(* Logix 5000 AddOnInstructionDefinition export Banner_R95C8UI_Param_v4; software revision 33.00 *)

TYPE Banner_IOL_Port_v4 :   // UDT that has all of the data items necessary to communicate with a specific Port on a IO-Link Master
STRUCT
   Port_Controlled : INT;   // Each bit represents a port on an IO-Link Master. Set to 1 to tell AOI to control that port.
   Port_Activate : INT;   // Each bit represents a port on an IO-Link Master. When ON that port will process any commands in queue.
   Port_Read : INT;   // Each bit represents a port on an IO-Link Master. Used to determine when device AOI has requested a Read command.
   Port_Write : INT;   // Each bit represents a port on an IO-Link Master. Used to determine when device AOI has requested a Write command.
   Port_RW_Complete : INT;   // Each bit represents a port on an IO-Link Master. Tells device AOI that Read or Write request has been completed.
   Port_Device_Read : INT;
   Data_Transfer : SINT[190];   // Array to transfer data from IO-Master to device AOIs.
END_STRUCT
END_TYPE

TYPE Banner_R95C_8UI_MDC_v4 :   // MDC Descriptor parameters for Smart Sensor Profile 2nd edition.
STRUCT
   Lower_Limit : DINT;
   Upper_Limit : DINT;
   Unit : INT;   // 1209 = A, 1240 = V
   Scale : SINT;
END_STRUCT
END_TYPE

TYPE Banner_R95C_8UI_RD_v4 :   // UDT that stores the Read Data for a R95C-8UI-KQ.
STRUCT
   Master_Cycle_Time : INT;
   Min_Cycle_Time : INT;
   M_Sequence_Capability : INT;
   IO_Link_Version_ID : INT;
   Process_Data_Input_Length : INT;
   Process_Data_Output_Length : INT;
   Combined_Vendor_ID : DINT;   // IO-Link Vendor ID
   Vendor_ID1 : INT;
   Vendor_ID2 : INT;
   Combined_Device_ID : DINT;   // IO-Link Device ID
   Device_ID1 : INT;
   Device_ID2 : INT;
   Device_ID3 : INT;
   Serial_Number : STRING;
   All_Time_Run_Time : DINT;
   MDC : Banner_R95C_8UI_MDC_v4[9];
END_STRUCT
END_TYPE

TYPE Banner_R95C_8UI_Setpoints_v4 :   // The Channel setpoints for a R95C-8UI-KQ.
STRUCT
   Voltage_SP1 : DINT;   // Lower limit setpoint.
   Voltage_SP2 : DINT;   // Upper limit setpoint.
   Voltage_Hysteresis : DINT;   // Hysteresis value for the voltage switchpont.
   Current_SP1 : DINT;   // Lower limit setpoint.
   Current_SP2 : DINT;   // Upper limit setpoint.
   Current_Hysteresis : DINT;   // Hysteresis value for the current switchpont.
END_STRUCT
END_TYPE

TYPE Banner_R95C_8UI_v4 :   // All of the parameters for a R95C-8UI-KQ.
STRUCT
   Initial_Global_Read : BOOL;   // Determines if all of the IO-Link data has been read into the PLC yet
   Command : INT;   // Value placed in here will activate a read or write to a specifc IO-Link Index
   Read : Banner_R95C_8UI_RD_v4;   // Read Only Data
   Write : Banner_R95C_8UI_WD_v4;   // Write Data
   Archive : Banner_R95C_8UI_WD_v4;   // Archive of the Write Data
   Reset : BOOL;   // Resets AOI. This will force a complete parameter read of the sensor.
END_STRUCT
END_TYPE

TYPE Banner_R95C_8UI_VSC_v4 :   // Vendor Specific Configuration data elements for a R95C-8UI-KQ.
STRUCT
   PDI_Config : SINT;   // 0 = Analog Value, 1 = Digital Measuring Sensor.
   IOL_Filter_Time : INT;   // Timer to average IOL process data measurement between updates.
   Secondary_Output_Function : SINT;   // 0 = Disabled, 1 = Puse Frequency Modulation.
   PFM_Input_Port : SINT;   // 0 = Analog 1, 1 = Analog 2, 2= Analog 3, 3 = Analog 4, 4 = Analog 5, 5 = Analog 6, 6 = Analog 7, 7 = Analog 8.
   Analog_1_Mode : SINT;   // 0 = Voltage, 1 = Current.
   Analog_2_Mode : SINT;   // 0 = Voltage, 1 = Current.
   Analog_3_Mode : SINT;   // 0 = Voltage, 1 = Current.
   Analog_4_Mode : SINT;   // 0 = Voltage, 1 = Current.
   Analog_5_Mode : SINT;   // 0 = Voltage, 1 = Current.
   Analog_6_Mode : SINT;   // 0 = Voltage, 1 = Current.
   Analog_7_Mode : SINT;   // 0 = Voltage, 1 = Current.
   Analog_8_Mode : SINT;   // 0 = Voltage, 1 = Current.
END_STRUCT
END_TYPE

TYPE Banner_R95C_8UI_WD_v4 :   // UDT that stores the Write Data for a R95C-8UI-KQ.
STRUCT
   System_Command : INT;   // See IODD file for list of commands that can be activated via the System Command interface
   Parameter_Access_Lock : SINT;   // Write access to all parameters is prohibited while value is 1. Only this parameter can be adjusted when value is 1.
   Data_Storage_Lock : SINT;   // Automatic data storage is disabled when this value is equal to 1. Read access is not affected.
   Local_Parameterization_Lock : SINT;   // Parameterization via local control elements on device is disabled.
   Local_User_Interface_Lock : SINT;   // Operation of local user interface is disabled.
   Resettable_Run_Time : DINT;   // Read/Write time counter in hours.
   Near_Freq : DINT;   // 100 to 45000 Hz.
   Far_Freq : DINT;   // 100 to 45000 Hz.
   Pulse_Freq_LOS : DINT;   // 50. Value that the Pulse frequency defaults to when a loss of signal occurs.
   VSC : Banner_R95C_8UI_VSC_v4;
   All_Time_Run_Time_Event_Time : DINT;   // Event indicating the corresponding configured running time has elapsed.
   Resettable_Run_Time_Event_TIme : DINT;   // Running time when an event will be raised indicating that service is required.
   Setpoints : Banner_R95C_8UI_Setpoints_v4[9];
END_STRUCT
END_TYPE

ADD_ON_INSTRUCTION Banner_R95C8UI_Param_v4   (* revision 4.0, vendor Banner Engineering *)
// AOI to read and write parameter data to an IO-Link R95C-8UI-KQ.
VAR_IN_OUT
   R95C : Banner_R95C_8UI_v4; {required}
   Port_Data : Banner_IOL_Port_v4; {required}
END_VAR
VAR_INPUT
   Port : INT; {required}   // Port Number that device is plugged into.
END_VAR
VAR
   Local_Control : DINT; {access None}
   Global_Read_Command_Value : INT; {access None}
   Global_Write_Command_Value : INT; {access None}
   Command_Being_Processed : BOOL; {access None}
   Update_Archive : BOOL; {access None}
   Index_Write_Inprocess : DINT; {access None}
   Index_Write_Control : DINT; {access None}
   Inprocess_Index : DINT; {access None}
   Index1 : DINT; {access None}
   Index2 : DINT; {access None}
   Index3 : DINT; {access None}
   Index_Segment_Read : DINT; {access None}
END_VAR

ROUTINE Logic   (* ladder *)
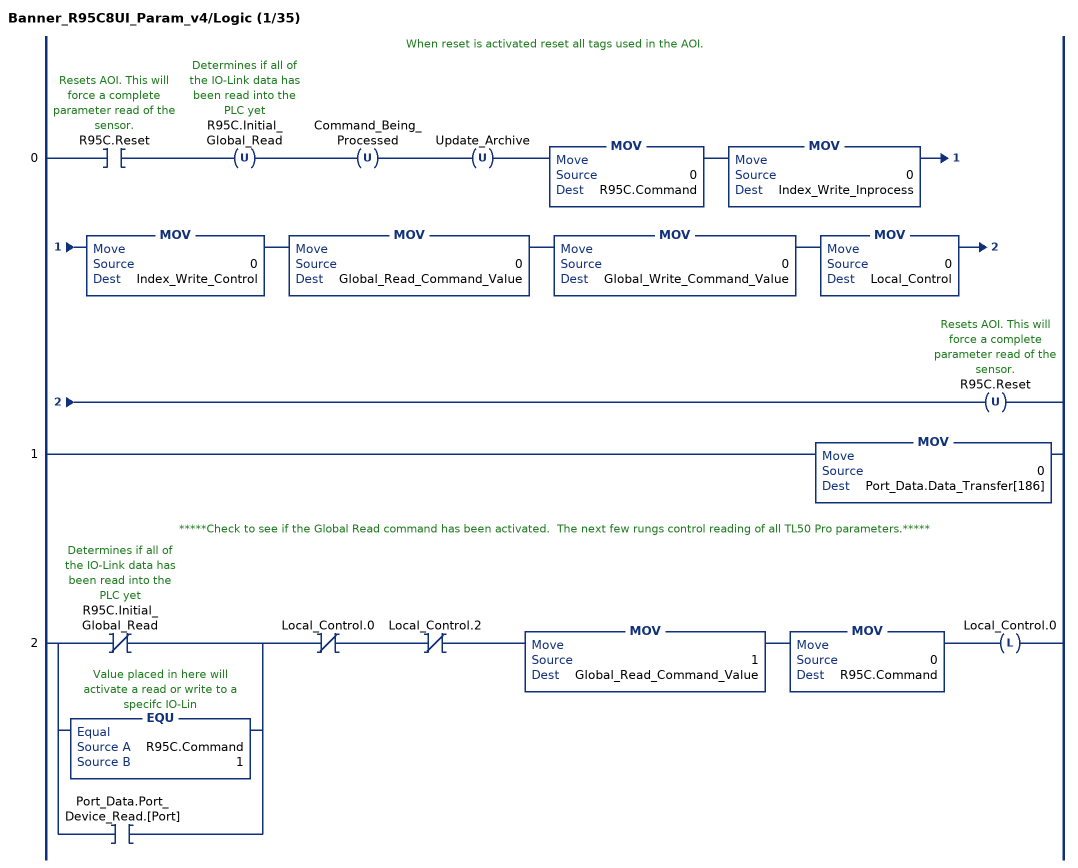
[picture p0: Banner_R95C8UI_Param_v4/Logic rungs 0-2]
   // When reset is activated reset all tags used in the AOI.
   0: XIC(R95C.Reset)OTU(R95C.Initial_Global_Read)OTU(Command_Being_Processed)OTU(Update_Archive)MOV(0,R95C.Command)MOV(0,Index_Write_Inprocess)MOV(0,Index_Write_Control)MOV(0,Global_Read_Command_Value)MOV(0,Global_Write_Command_Value)MOV(0,Local_Control)OTU(R95C.Reset);
   1: MOV(0,Port_Data.Data_Transfer[186]);
   // *****Check to see if the Global Read command has been activated.  The next few rungs control reading of all TL50 Pro parameters.*****
   2: [XIO(R95C.Initial_Global_Read) ,EQU(R95C.Command,1) ,XIC(Port_Data.Port_Device_Read.[Port]) ]XIO(Local_Control.0)XIO(Local_Control.2)MOV(1,Global_Read_Command_Value)MOV(0,R95C.Command)OTL(Local_Control.0);
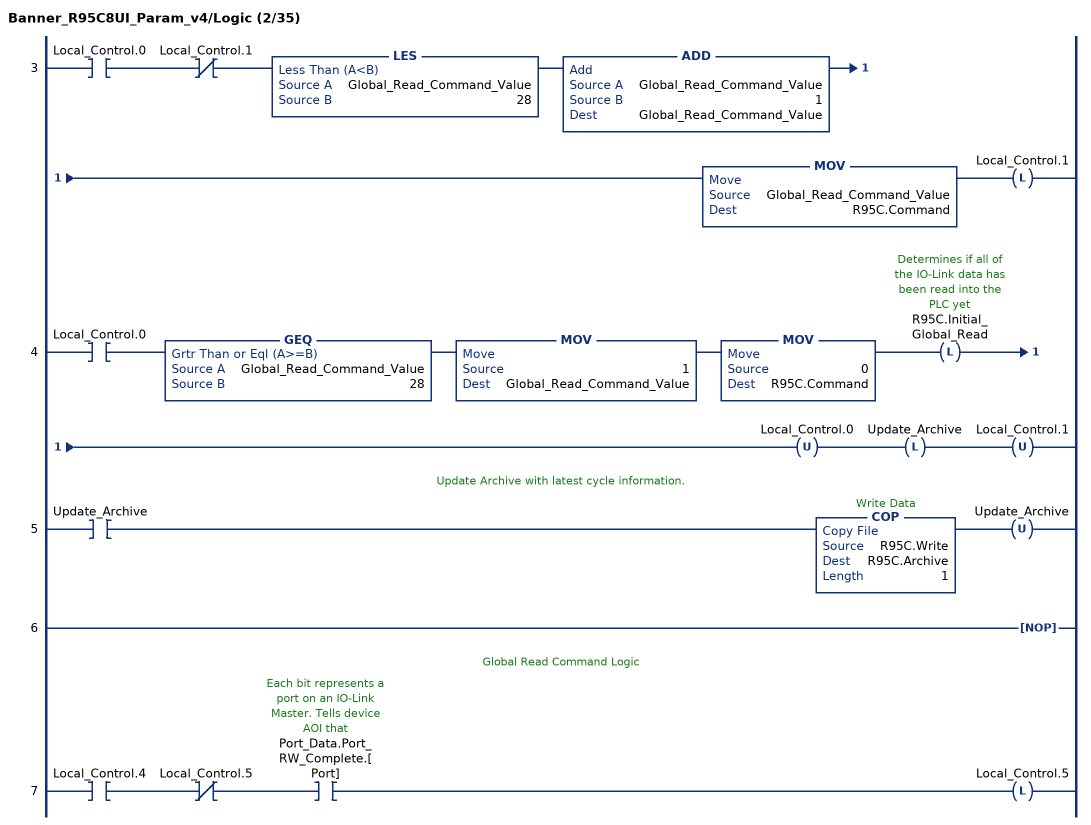
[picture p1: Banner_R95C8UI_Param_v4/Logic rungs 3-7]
   3: XIC(Local_Control.0)XIO(Local_Control.1)LES(Global_Read_Command_Value,28)ADD(Global_Read_Command_Value,1,Global_Read_Command_Value)MOV(Global_Read_Command_Value,R95C.Command)OTL(Local_Control.1);
   4: XIC(Local_Control.0)GEQ(Global_Read_Command_Value,28)MOV(1,Global_Read_Command_Value)MOV(0,R95C.Command)OTL(R95C.Initial_Global_Read)OTU(Local_Control.0)OTL(Update_Archive)OTU(Local_Control.1);
   // Update Archive with latest cycle information.
   5: XIC(Update_Archive)COP(R95C.Write,R95C.Archive,1)OTU(Update_Archive);
   6: NOP();
   // Global Read Command Logic
   7: XIC(Local_Control.4)XIO(Local_Control.5)XIC(Port_Data.Port_RW_Complete.[Port])OTL(Local_Control.5);
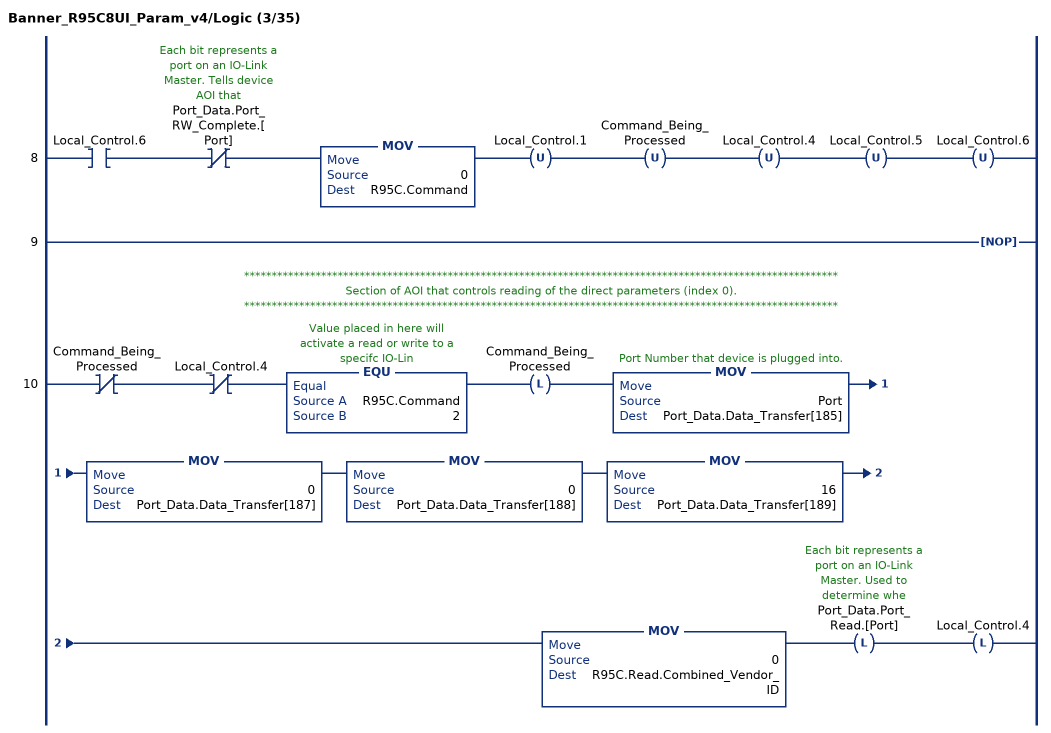
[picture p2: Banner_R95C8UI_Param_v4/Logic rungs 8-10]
   8: XIC(Local_Control.6)XIO(Port_Data.Port_RW_Complete.[Port])MOV(0,R95C.Command)OTU(Local_Control.1)OTU(Command_Being_Processed)OTU(Local_Control.4)OTU(Local_Control.5)OTU(Local_Control.6);
   9: NOP();
   // ************************************************************************************************************
   // Section of AOI that controls reading of the direct parameters (index 0).
   // ************************************************************************************************************
   10: XIO(Command_Being_Processed)XIO(Local_Control.4)EQU(R95C.Command,2)OTL(Command_Being_Processed)MOV(Port,Port_Data.Data_Transfer[185])MOV(0,Port_Data.Data_Transfer[187])MOV(0,Port_Data.Data_Transfer[188])MOV(16,Port_Data.Data_Transfer[189])MOV(0,R95C.Read.Combined_Vendor_ID)OTL(Port_Data.Port_Read.[Port])OTL(Local_Control.4);
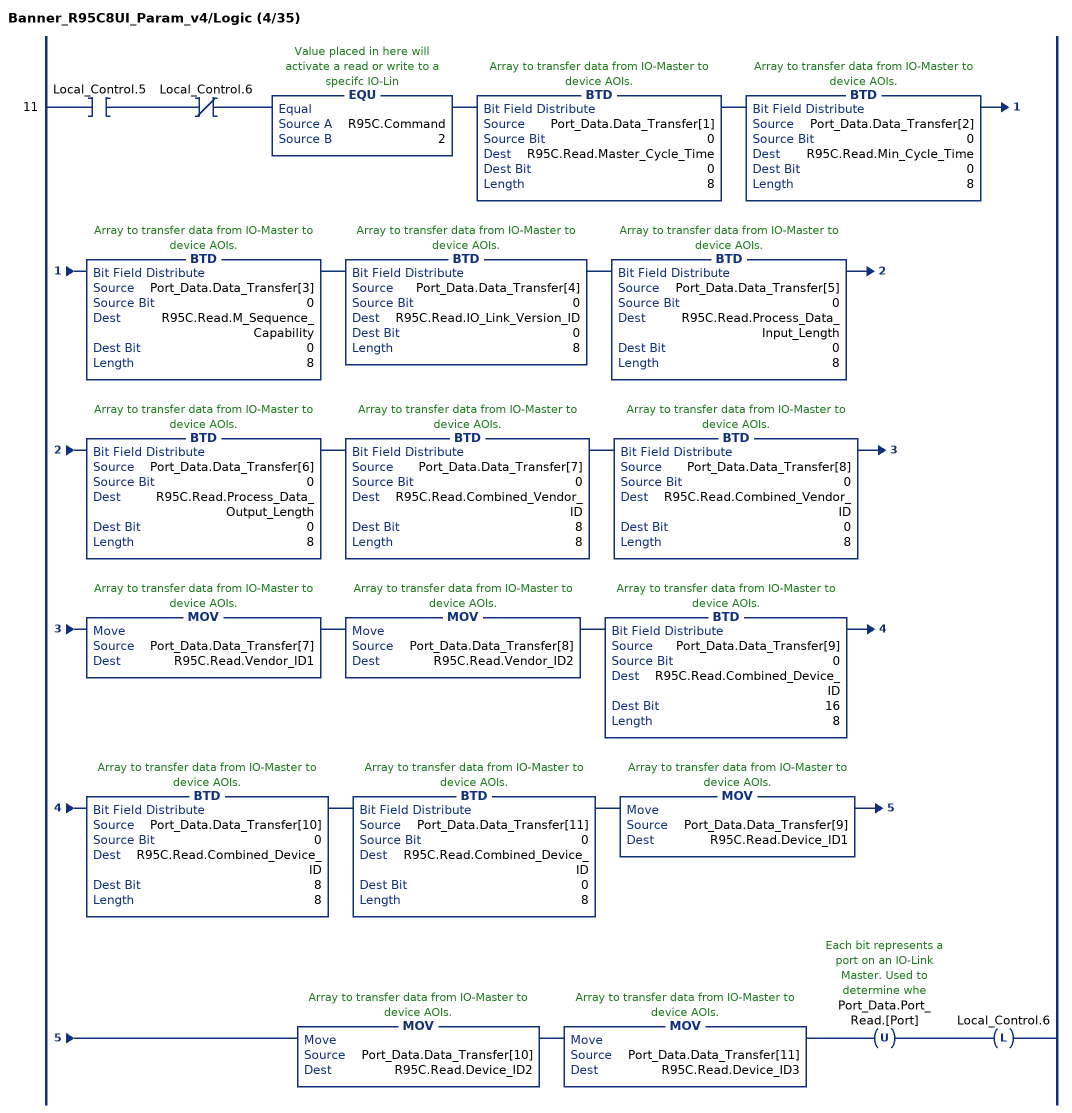
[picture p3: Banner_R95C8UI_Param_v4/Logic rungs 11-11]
   11: XIC(Local_Control.5)XIO(Local_Control.6)EQU(R95C.Command,2)BTD(Port_Data.Data_Transfer[1],0,R95C.Read.Master_Cycle_Time,0,8)BTD(Port_Data.Data_Transfer[2],0,R95C.Read.Min_Cycle_Time,0,8)BTD(Port_Data.Data_Transfer[3],0,R95C.Read.M_Sequence_Capability,0,8)BTD(Port_Data.Data_Transfer[4],0,R95C.Read.IO_Link_Version_ID,0,8)BTD(Port_Data.Data_Transfer[5],0,R95C.Read.Process_Data_Input_Length,0,8)BTD(Port_Data.Data_Transfer[6],0,R95C.Read.Process_Data_Output_Length,0,8)BTD(Port_Data.Data_Transfer[7],0,R95C.Read.Combined_Vendor_ID,8,8)BTD(Port_Data.Data_Transfer[8],0,R95C.Read.Combined_Vendor_ID,0,8)MOV(Port_Data.Data_Transfer[7],R95C.Read.Vendor_ID1)MOV(Port_Data.Data_Transfer[8],R95C.Read.Vendor_ID2)BTD(Port_Data.Data_Transfer[9],0,R95C.Read.Combined_Device_ID,16,8)BTD(Port_Data.Data_Transfer[10],0,R95C.Read.Combined_Device_ID,8,8)BTD(Port_Data.Data_Transfer[11],0,R95C.Read.Combined_Device_ID,0,8)MOV(Port_Data.Data_Transfer[9],R95C.Read.Device_ID1)MOV(Port_Data.Data_Transfer[10],R95C.Read.Device_ID2)MOV(Port_Data.Data_Transfer[11],R95C.Read.Device_ID3)OTU(Port_Data.Port_Read.[Port])OTL(Local_Control.6);
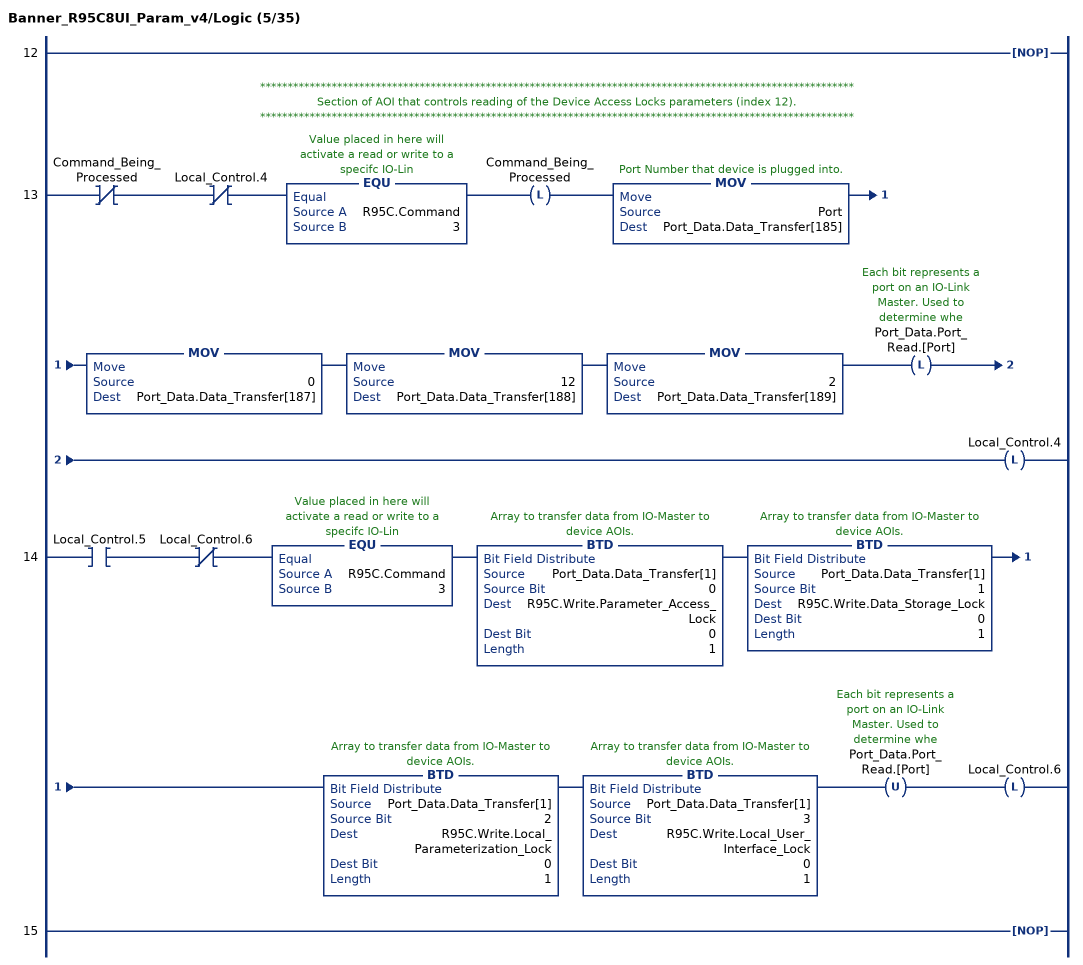
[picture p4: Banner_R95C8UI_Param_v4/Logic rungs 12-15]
   12: NOP();
   // ************************************************************************************************************
   // Section of AOI that controls reading of the Device Access Locks parameters (index 12).
   // ************************************************************************************************************
   13: XIO(Command_Being_Processed)XIO(Local_Control.4)EQU(R95C.Command,3)OTL(Command_Being_Processed)MOV(Port,Port_Data.Data_Transfer[185])MOV(0,Port_Data.Data_Transfer[187])MOV(12,Port_Data.Data_Transfer[188])MOV(2,Port_Data.Data_Transfer[189])OTL(Port_Data.Port_Read.[Port])OTL(Local_Control.4);
   14: XIC(Local_Control.5)XIO(Local_Control.6)EQU(R95C.Command,3)BTD(Port_Data.Data_Transfer[1],0,R95C.Write.Parameter_Access_Lock,0,1)BTD(Port_Data.Data_Transfer[1],1,R95C.Write.Data_Storage_Lock,0,1)BTD(Port_Data.Data_Transfer[1],2,R95C.Write.Local_Parameterization_Lock,0,1)BTD(Port_Data.Data_Transfer[1],3,R95C.Write.Local_User_Interface_Lock,0,1)OTU(Port_Data.Port_Read.[Port])OTL(Local_Control.6);
   15: NOP();
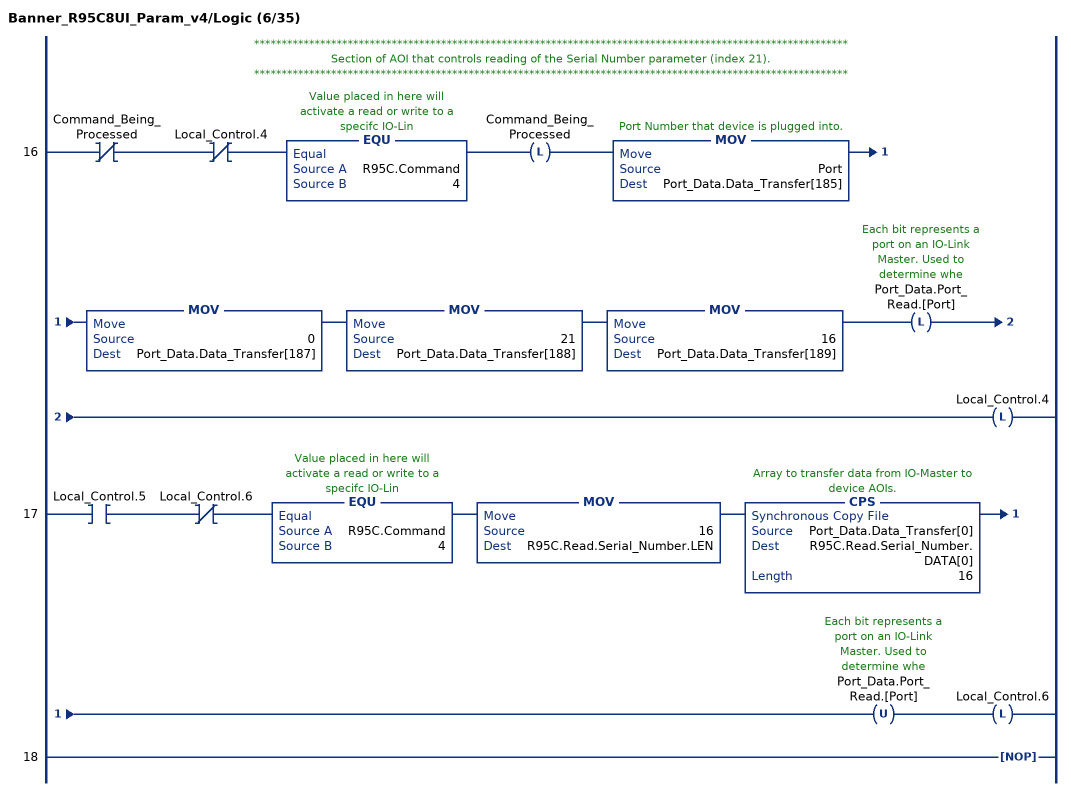
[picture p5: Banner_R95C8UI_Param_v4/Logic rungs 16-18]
   // ************************************************************************************************************
   // Section of AOI that controls reading of the Serial Number parameter (index 21).
   // ************************************************************************************************************
   16: XIO(Command_Being_Processed)XIO(Local_Control.4)EQU(R95C.Command,4)OTL(Command_Being_Processed)MOV(Port,Port_Data.Data_Transfer[185])MOV(0,Port_Data.Data_Transfer[187])MOV(21,Port_Data.Data_Transfer[188])MOV(16,Port_Data.Data_Transfer[189])OTL(Port_Data.Port_Read.[Port])OTL(Local_Control.4);
   17: XIC(Local_Control.5)XIO(Local_Control.6)EQU(R95C.Command,4)MOV(16,R95C.Read.Serial_Number.LEN)CPS(Port_Data.Data_Transfer[0],R95C.Read.Serial_Number.DATA[0],16)OTU(Port_Data.Port_Read.[Port])OTL(Local_Control.6);
   18: NOP();
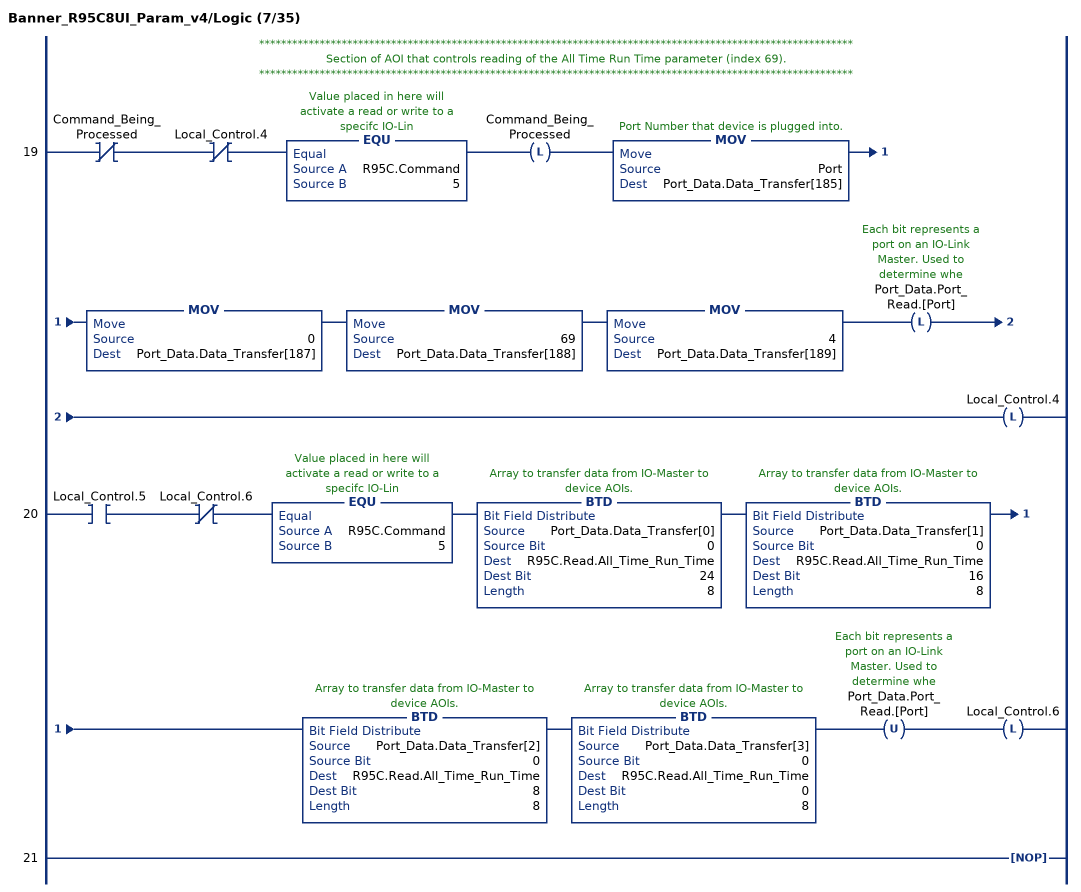
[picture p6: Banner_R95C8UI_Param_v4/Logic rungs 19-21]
   // ************************************************************************************************************
   // Section of AOI that controls reading of the All Time Run Time parameter (index 69).
   // ************************************************************************************************************
   19: XIO(Command_Being_Processed)XIO(Local_Control.4)EQU(R95C.Command,5)OTL(Command_Being_Processed)MOV(Port,Port_Data.Data_Transfer[185])MOV(0,Port_Data.Data_Transfer[187])MOV(69,Port_Data.Data_Transfer[188])MOV(4,Port_Data.Data_Transfer[189])OTL(Port_Data.Port_Read.[Port])OTL(Local_Control.4);
   20: XIC(Local_Control.5)XIO(Local_Control.6)EQU(R95C.Command,5)BTD(Port_Data.Data_Transfer[0],0,R95C.Read.All_Time_Run_Time,24,8)BTD(Port_Data.Data_Transfer[1],0,R95C.Read.All_Time_Run_Time,16,8)BTD(Port_Data.Data_Transfer[2],0,R95C.Read.All_Time_Run_Time,8,8)BTD(Port_Data.Data_Transfer[3],0,R95C.Read.All_Time_Run_Time,0,8)OTU(Port_Data.Port_Read.[Port])OTL(Local_Control.6);
   21: NOP();
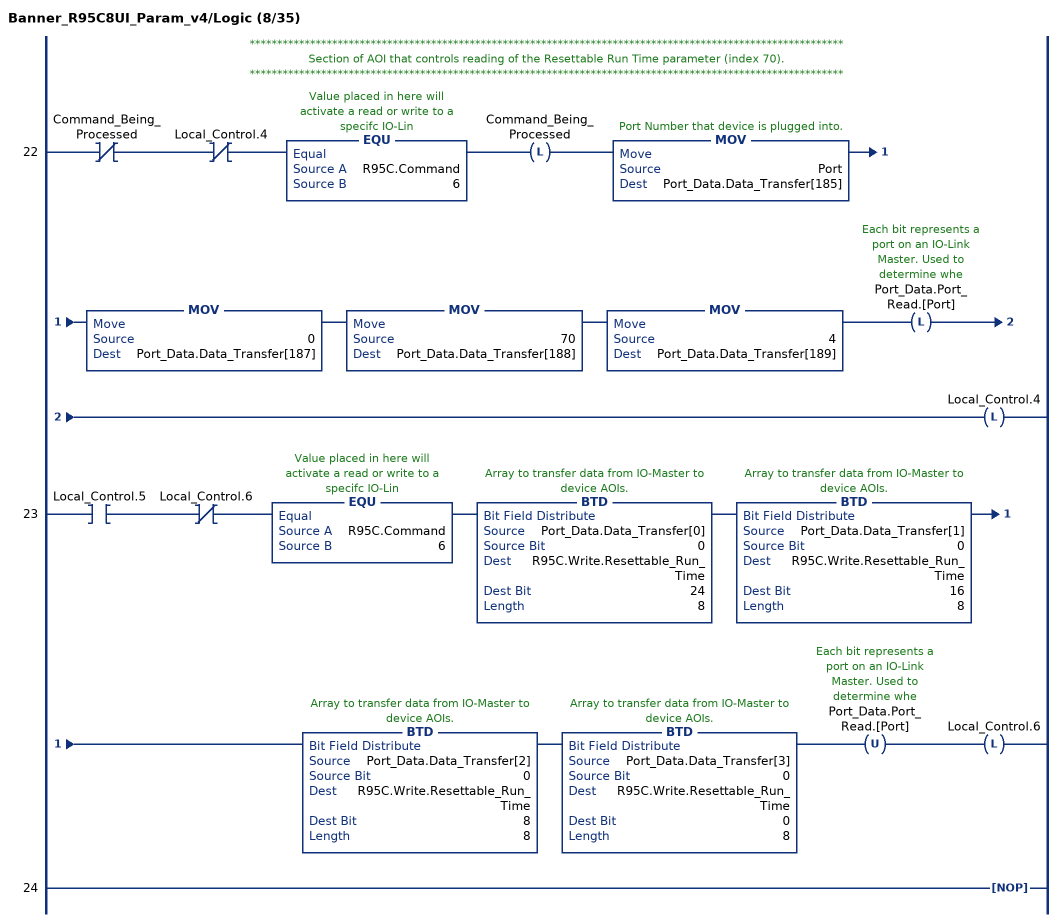
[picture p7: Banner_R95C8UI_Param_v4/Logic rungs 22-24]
   // ************************************************************************************************************
   // Section of AOI that controls reading of the Resettable Run Time parameter (index 70).
   // ************************************************************************************************************
   22: XIO(Command_Being_Processed)XIO(Local_Control.4)EQU(R95C.Command,6)OTL(Command_Being_Processed)MOV(Port,Port_Data.Data_Transfer[185])MOV(0,Port_Data.Data_Transfer[187])MOV(70,Port_Data.Data_Transfer[188])MOV(4,Port_Data.Data_Transfer[189])OTL(Port_Data.Port_Read.[Port])OTL(Local_Control.4);
   23: XIC(Local_Control.5)XIO(Local_Control.6)EQU(R95C.Command,6)BTD(Port_Data.Data_Transfer[0],0,R95C.Write.Resettable_Run_Time,24,8)BTD(Port_Data.Data_Transfer[1],0,R95C.Write.Resettable_Run_Time,16,8)BTD(Port_Data.Data_Transfer[2],0,R95C.Write.Resettable_Run_Time,8,8)BTD(Port_Data.Data_Transfer[3],0,R95C.Write.Resettable_Run_Time,0,8)OTU(Port_Data.Port_Read.[Port])OTL(Local_Control.6);
   24: NOP();
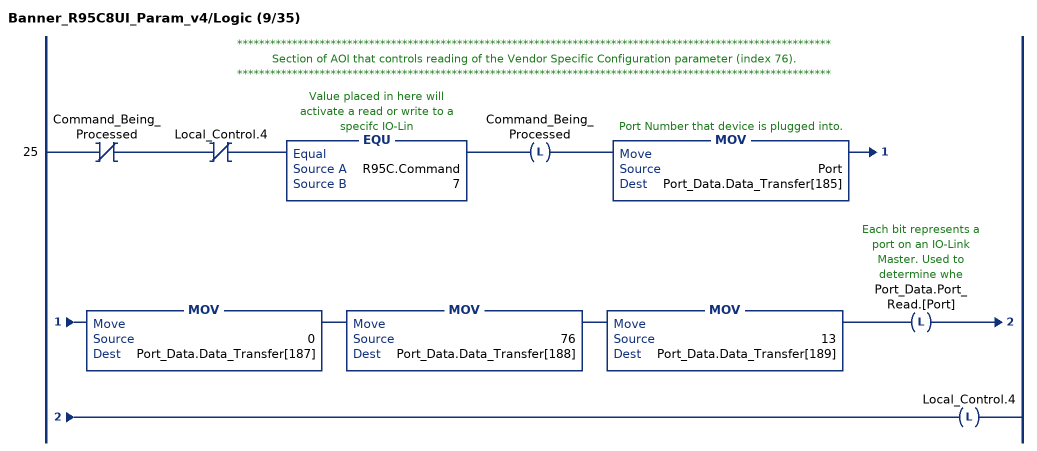
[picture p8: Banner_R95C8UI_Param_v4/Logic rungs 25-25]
   // ************************************************************************************************************
   // Section of AOI that controls reading of the Vendor Specific Configuration parameter (index 76).
   // ************************************************************************************************************
   25: XIO(Command_Being_Processed)XIO(Local_Control.4)EQU(R95C.Command,7)OTL(Command_Being_Processed)MOV(Port,Port_Data.Data_Transfer[185])MOV(0,Port_Data.Data_Transfer[187])MOV(76,Port_Data.Data_Transfer[188])MOV(13,Port_Data.Data_Transfer[189])OTL(Port_Data.Port_Read.[Port])OTL(Local_Control.4);
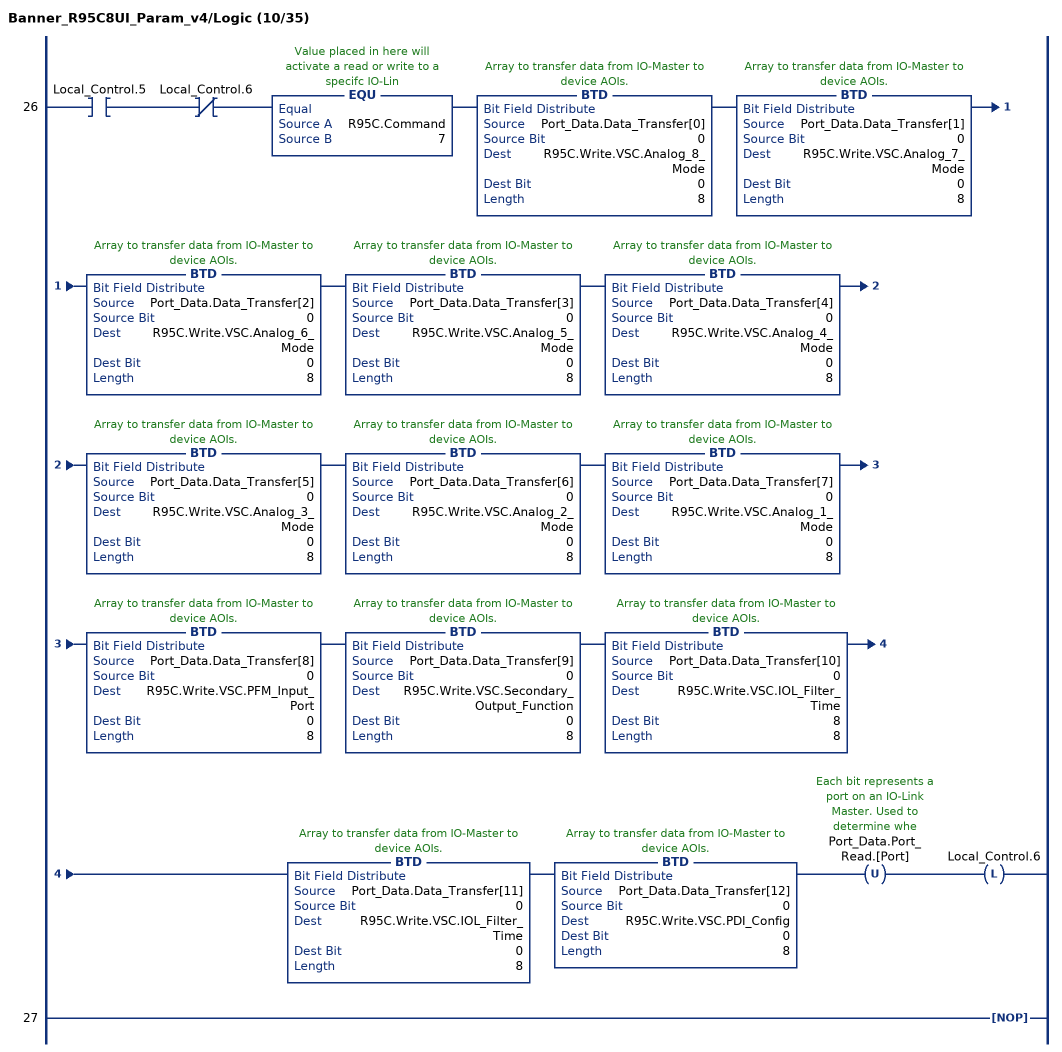
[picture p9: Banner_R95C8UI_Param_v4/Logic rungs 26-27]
   26: XIC(Local_Control.5)XIO(Local_Control.6)EQU(R95C.Command,7)BTD(Port_Data.Data_Transfer[0],0,R95C.Write.VSC.Analog_8_Mode,0,8)BTD(Port_Data.Data_Transfer[1],0,R95C.Write.VSC.Analog_7_Mode,0,8)BTD(Port_Data.Data_Transfer[2],0,R95C.Write.VSC.Analog_6_Mode,0,8)BTD(Port_Data.Data_Transfer[3],0,R95C.Write.VSC.Analog_5_Mode,0,8)BTD(Port_Data.Data_Transfer[4],0,R95C.Write.VSC.Analog_4_Mode,0,8)BTD(Port_Data.Data_Transfer[5],0,R95C.Write.VSC.Analog_3_Mode,0,8)BTD(Port_Data.Data_Transfer[6],0,R95C.Write.VSC.Analog_2_Mode,0,8)BTD(Port_Data.Data_Transfer[7],0,R95C.Write.VSC.Analog_1_Mode,0,8)BTD(Port_Data.Data_Transfer[8],0,R95C.Write.VSC.PFM_Input_Port,0,8)BTD(Port_Data.Data_Transfer[9],0,R95C.Write.VSC.Secondary_Output_Function,0,8)BTD(Port_Data.Data_Transfer[10],0,R95C.Write.VSC.IOL_Filter_Time,8,8)BTD(Port_Data.Data_Transfer[11],0,R95C.Write.VSC.IOL_Filter_Time,0,8)BTD(Port_Data.Data_Transfer[12],0,R95C.Write.VSC.PDI_Config,0,8)OTU(Port_Data.Port_Read.[Port])OTL(Local_Control.6);
   27: NOP();
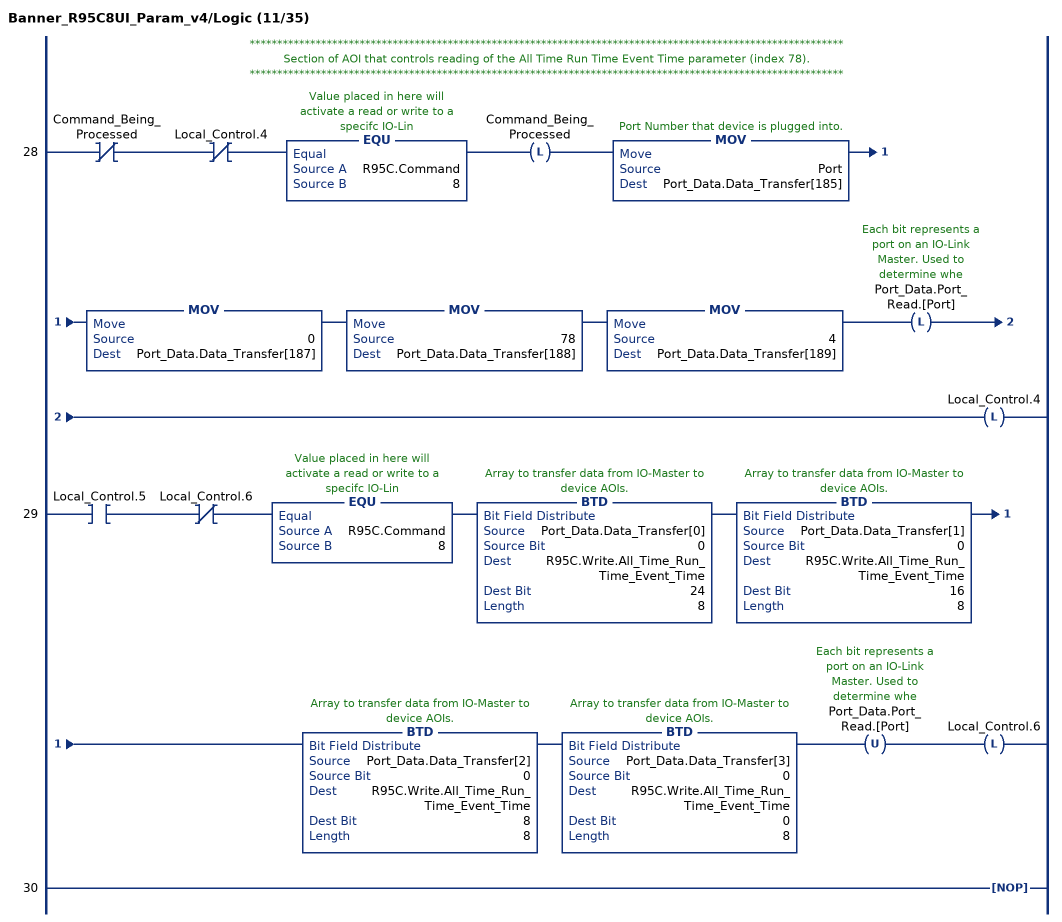
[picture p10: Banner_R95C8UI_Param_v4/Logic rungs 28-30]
   // ************************************************************************************************************
   // Section of AOI that controls reading of the All Time Run Time Event Time parameter (index 78).
   // ************************************************************************************************************
   28: XIO(Command_Being_Processed)XIO(Local_Control.4)EQU(R95C.Command,8)OTL(Command_Being_Processed)MOV(Port,Port_Data.Data_Transfer[185])MOV(0,Port_Data.Data_Transfer[187])MOV(78,Port_Data.Data_Transfer[188])MOV(4,Port_Data.Data_Transfer[189])OTL(Port_Data.Port_Read.[Port])OTL(Local_Control.4);
   29: XIC(Local_Control.5)XIO(Local_Control.6)EQU(R95C.Command,8)BTD(Port_Data.Data_Transfer[0],0,R95C.Write.All_Time_Run_Time_Event_Time,24,8)BTD(Port_Data.Data_Transfer[1],0,R95C.Write.All_Time_Run_Time_Event_Time,16,8)BTD(Port_Data.Data_Transfer[2],0,R95C.Write.All_Time_Run_Time_Event_Time,8,8)BTD(Port_Data.Data_Transfer[3],0,R95C.Write.All_Time_Run_Time_Event_Time,0,8)OTU(Port_Data.Port_Read.[Port])OTL(Local_Control.6);
   30: NOP();
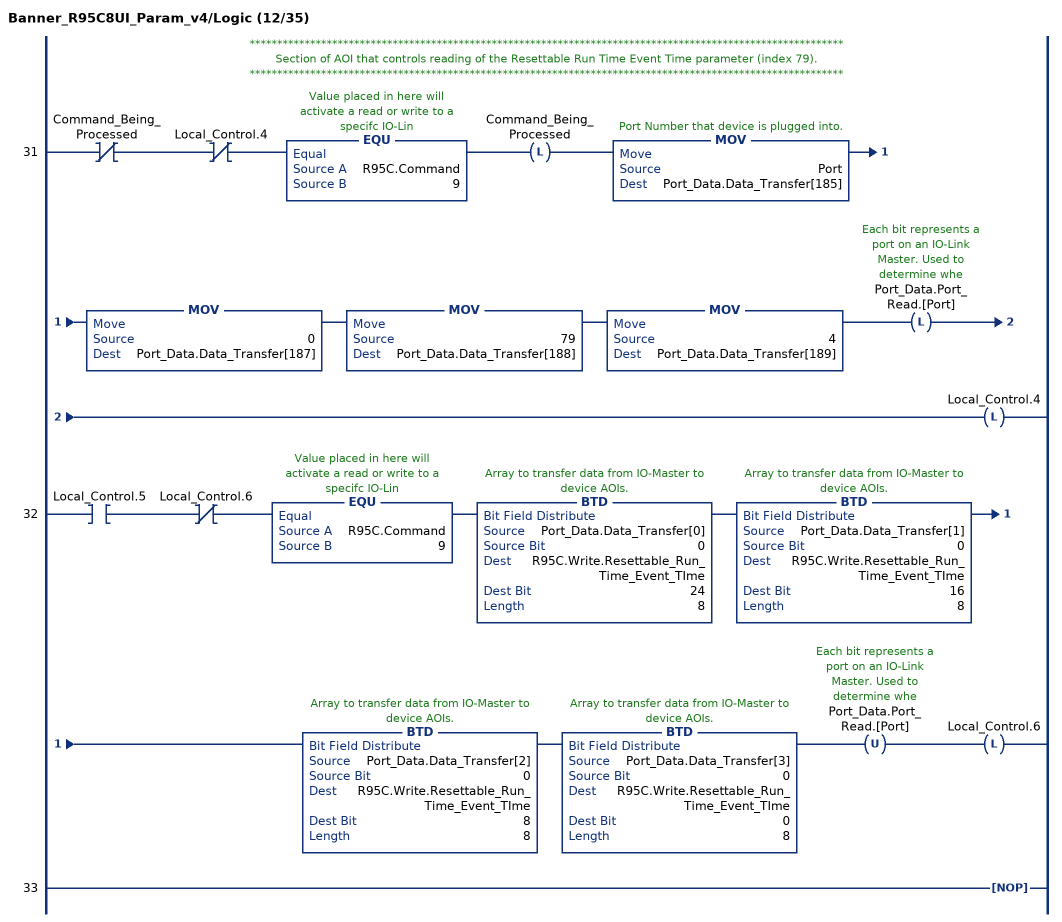
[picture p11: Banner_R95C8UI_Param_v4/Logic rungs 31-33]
   // ************************************************************************************************************
   // Section of AOI that controls reading of the Resettable Run Time Event Time parameter (index 79).
   // ************************************************************************************************************
   31: XIO(Command_Being_Processed)XIO(Local_Control.4)EQU(R95C.Command,9)OTL(Command_Being_Processed)MOV(Port,Port_Data.Data_Transfer[185])MOV(0,Port_Data.Data_Transfer[187])MOV(79,Port_Data.Data_Transfer[188])MOV(4,Port_Data.Data_Transfer[189])OTL(Port_Data.Port_Read.[Port])OTL(Local_Control.4);
   32: XIC(Local_Control.5)XIO(Local_Control.6)EQU(R95C.Command,9)BTD(Port_Data.Data_Transfer[0],0,R95C.Write.Resettable_Run_Time_Event_TIme,24,8)BTD(Port_Data.Data_Transfer[1],0,R95C.Write.Resettable_Run_Time_Event_TIme,16,8)BTD(Port_Data.Data_Transfer[2],0,R95C.Write.Resettable_Run_Time_Event_TIme,8,8)BTD(Port_Data.Data_Transfer[3],0,R95C.Write.Resettable_Run_Time_Event_TIme,0,8)OTU(Port_Data.Port_Read.[Port])OTL(Local_Control.6);
   33: NOP();
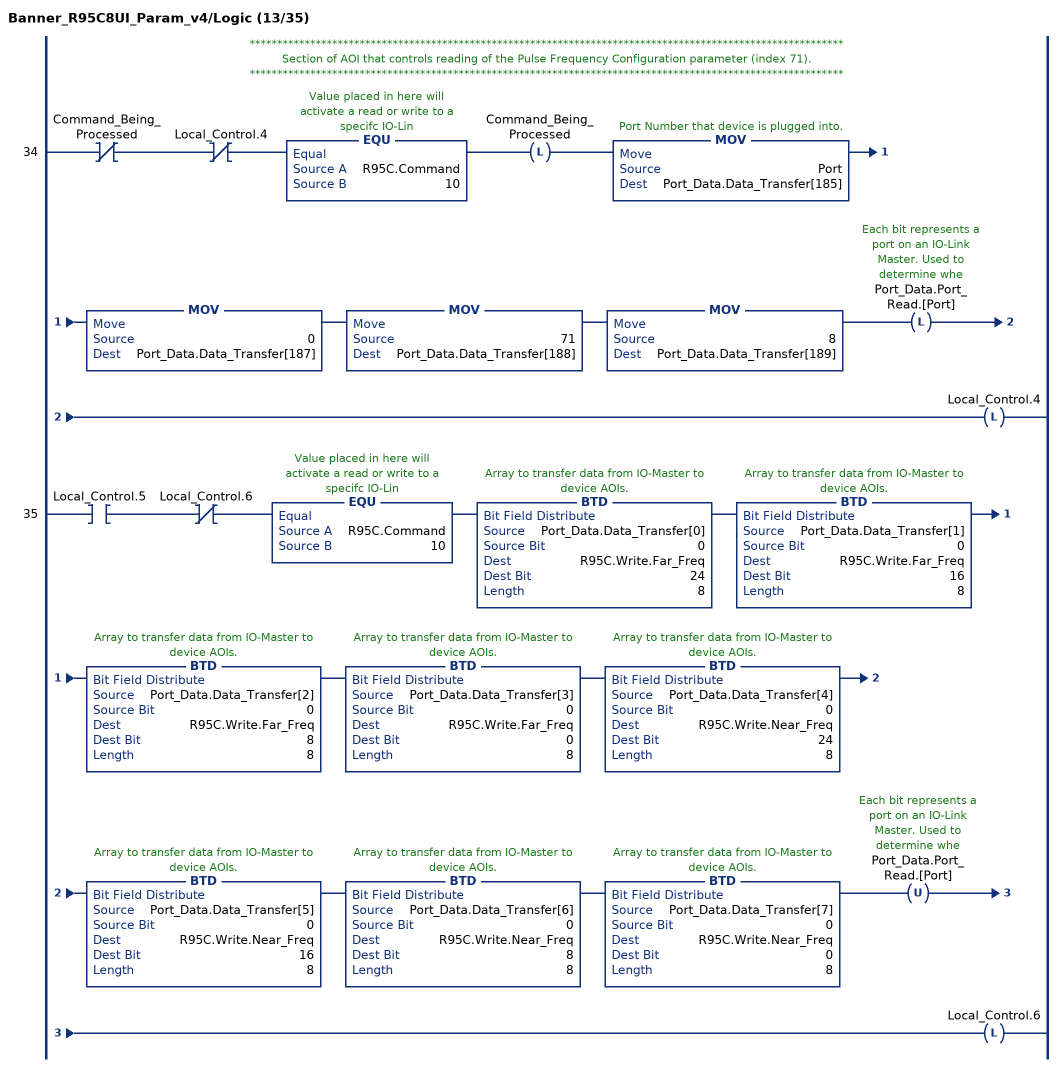
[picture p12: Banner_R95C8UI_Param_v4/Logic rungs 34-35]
   // ************************************************************************************************************
   // Section of AOI that controls reading of the Pulse Frequency Configuration parameter (index 71).
   // ************************************************************************************************************
   34: XIO(Command_Being_Processed)XIO(Local_Control.4)EQU(R95C.Command,10)OTL(Command_Being_Processed)MOV(Port,Port_Data.Data_Transfer[185])MOV(0,Port_Data.Data_Transfer[187])MOV(71,Port_Data.Data_Transfer[188])MOV(8,Port_Data.Data_Transfer[189])OTL(Port_Data.Port_Read.[Port])OTL(Local_Control.4);
   35: XIC(Local_Control.5)XIO(Local_Control.6)EQU(R95C.Command,10)BTD(Port_Data.Data_Transfer[0],0,R95C.Write.Far_Freq,24,8)BTD(Port_Data.Data_Transfer[1],0,R95C.Write.Far_Freq,16,8)BTD(Port_Data.Data_Transfer[2],0,R95C.Write.Far_Freq,8,8)BTD(Port_Data.Data_Transfer[3],0,R95C.Write.Far_Freq,0,8)BTD(Port_Data.Data_Transfer[4],0,R95C.Write.Near_Freq,24,8)BTD(Port_Data.Data_Transfer[5],0,R95C.Write.Near_Freq,16,8)BTD(Port_Data.Data_Transfer[6],0,R95C.Write.Near_Freq,8,8)BTD(Port_Data.Data_Transfer[7],0,R95C.Write.Near_Freq,0,8)OTU(Port_Data.Port_Read.[Port])OTL(Local_Control.6);
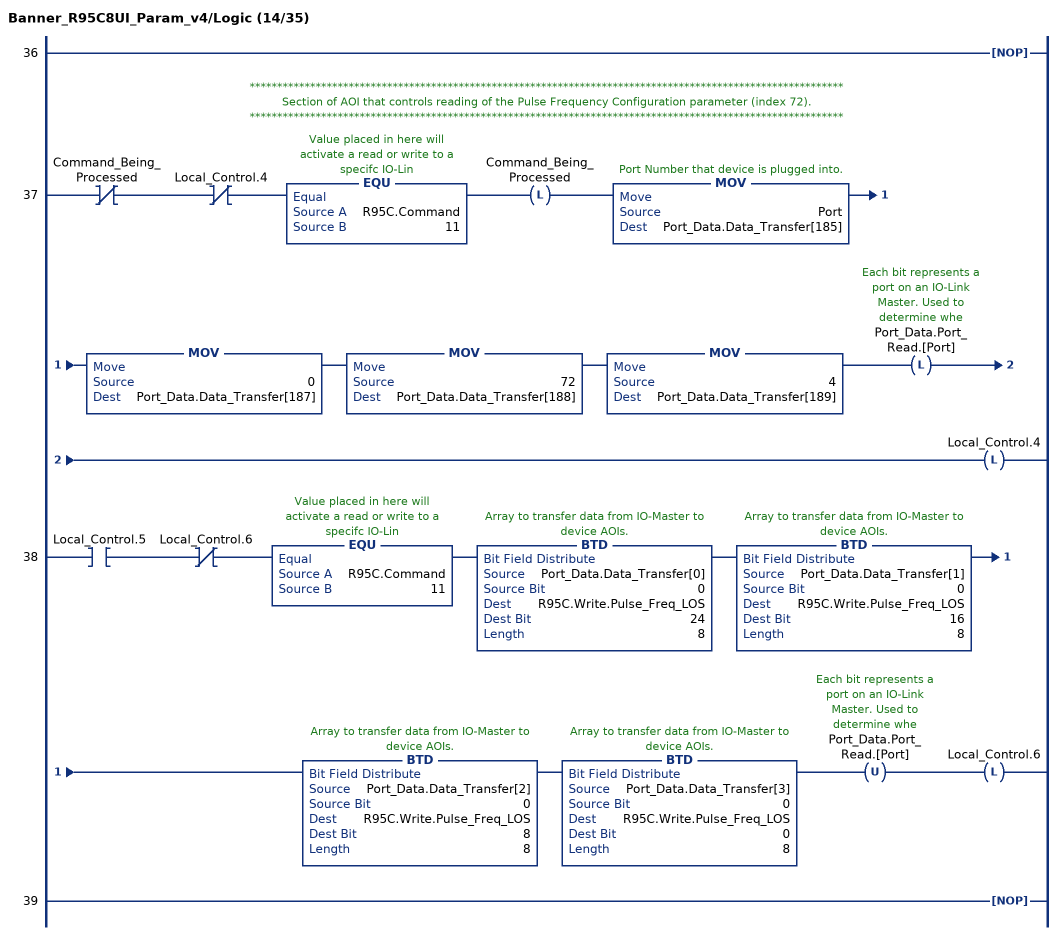
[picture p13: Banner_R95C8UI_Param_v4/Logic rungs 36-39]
   36: NOP();
   // ************************************************************************************************************
   // Section of AOI that controls reading of the Pulse Frequency Configuration parameter (index 72).
   // ************************************************************************************************************
   37: XIO(Command_Being_Processed)XIO(Local_Control.4)EQU(R95C.Command,11)OTL(Command_Being_Processed)MOV(Port,Port_Data.Data_Transfer[185])MOV(0,Port_Data.Data_Transfer[187])MOV(72,Port_Data.Data_Transfer[188])MOV(4,Port_Data.Data_Transfer[189])OTL(Port_Data.Port_Read.[Port])OTL(Local_Control.4);
   38: XIC(Local_Control.5)XIO(Local_Control.6)EQU(R95C.Command,11)BTD(Port_Data.Data_Transfer[0],0,R95C.Write.Pulse_Freq_LOS,24,8)BTD(Port_Data.Data_Transfer[1],0,R95C.Write.Pulse_Freq_LOS,16,8)BTD(Port_Data.Data_Transfer[2],0,R95C.Write.Pulse_Freq_LOS,8,8)BTD(Port_Data.Data_Transfer[3],0,R95C.Write.Pulse_Freq_LOS,0,8)OTU(Port_Data.Port_Read.[Port])OTL(Local_Control.6);
   39: NOP();
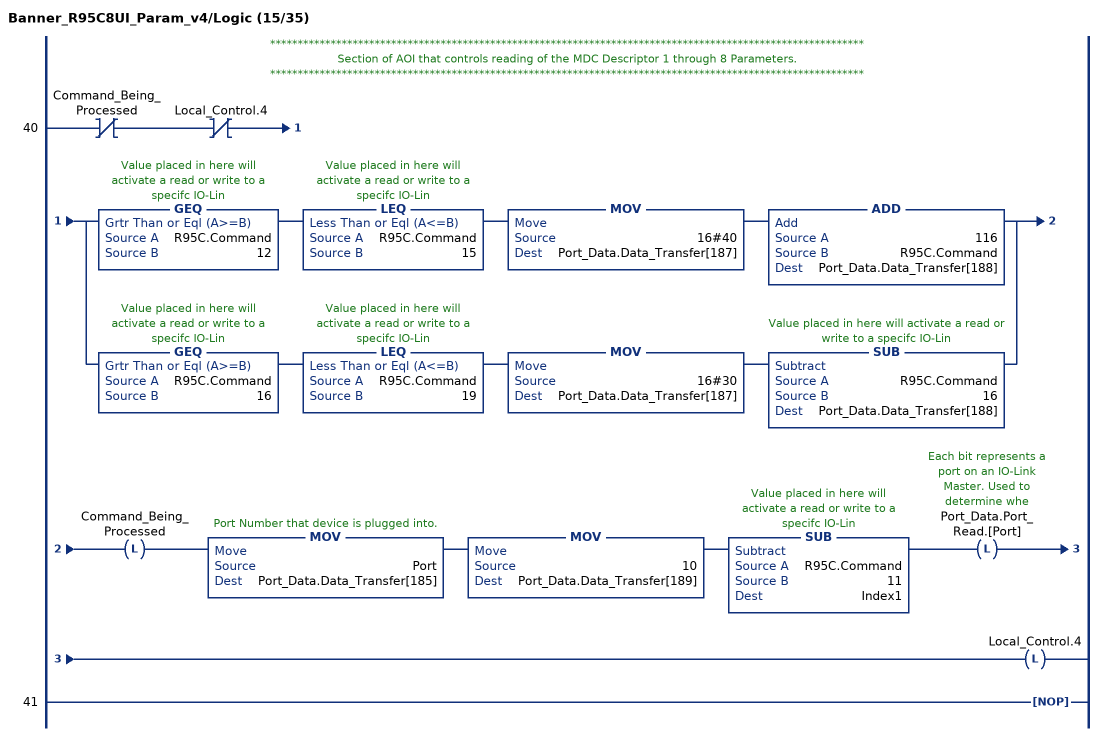
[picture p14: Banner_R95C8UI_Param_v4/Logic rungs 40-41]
   // ************************************************************************************************************
   // Section of AOI that controls reading of the MDC Descriptor 1 through 8 Parameters.
   // ************************************************************************************************************
   40: XIO(Command_Being_Processed)XIO(Local_Control.4)[GEQ(R95C.Command,12) LEQ(R95C.Command,15) MOV(16#40,Port_Data.Data_Transfer[187]) ADD(116,R95C.Command,Port_Data.Data_Transfer[188]) ,GEQ(R95C.Command,16) LEQ(R95C.Command,19) MOV(16#30,Port_Data.Data_Transfer[187]) SUB(R95C.Command,16,Port_Data.Data_Transfer[188]) ]OTL(Command_Being_Processed)MOV(Port,Port_Data.Data_Transfer[185])MOV(10,Port_Data.Data_Transfer[189])SUB(R95C.Command,11,Index1)OTL(Port_Data.Port_Read.[Port])OTL(Local_Control.4);
   41: NOP();
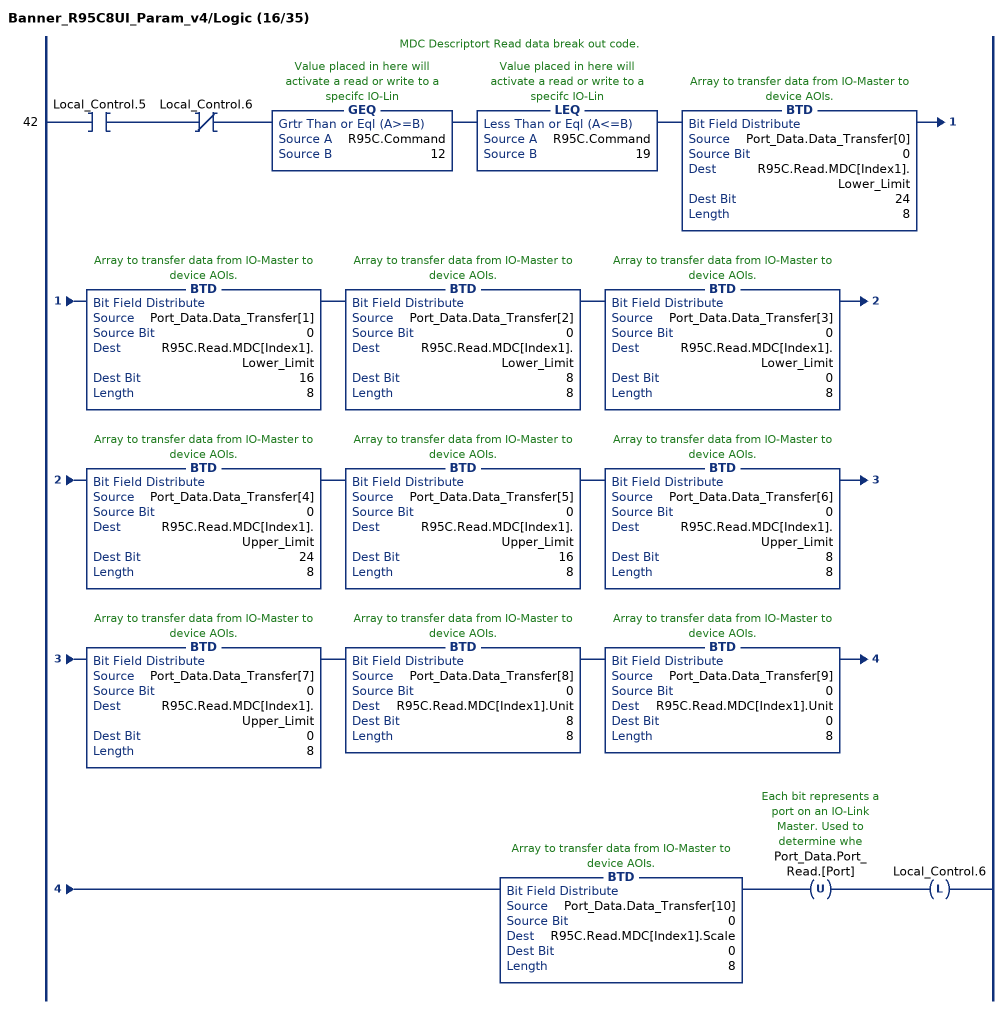
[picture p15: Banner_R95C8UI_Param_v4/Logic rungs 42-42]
   // MDC Descriptort Read data break out code.
   42: XIC(Local_Control.5)XIO(Local_Control.6)GEQ(R95C.Command,12)LEQ(R95C.Command,19)BTD(Port_Data.Data_Transfer[0],0,R95C.Read.MDC[Index1].Lower_Limit,24,8)BTD(Port_Data.Data_Transfer[1],0,R95C.Read.MDC[Index1].Lower_Limit,16,8)BTD(Port_Data.Data_Transfer[2],0,R95C.Read.MDC[Index1].Lower_Limit,8,8)BTD(Port_Data.Data_Transfer[3],0,R95C.Read.MDC[Index1].Lower_Limit,0,8)BTD(Port_Data.Data_Transfer[4],0,R95C.Read.MDC[Index1].Upper_Limit,24,8)BTD(Port_Data.Data_Transfer[5],0,R95C.Read.MDC[Index1].Upper_Limit,16,8)BTD(Port_Data.Data_Transfer[6],0,R95C.Read.MDC[Index1].Upper_Limit,8,8)BTD(Port_Data.Data_Transfer[7],0,R95C.Read.MDC[Index1].Upper_Limit,0,8)BTD(Port_Data.Data_Transfer[8],0,R95C.Read.MDC[Index1].Unit,8,8)BTD(Port_Data.Data_Transfer[9],0,R95C.Read.MDC[Index1].Unit,0,8)BTD(Port_Data.Data_Transfer[10],0,R95C.Read.MDC[Index1].Scale,0,8)OTU(Port_Data.Port_Read.[Port])OTL(Local_Control.6);
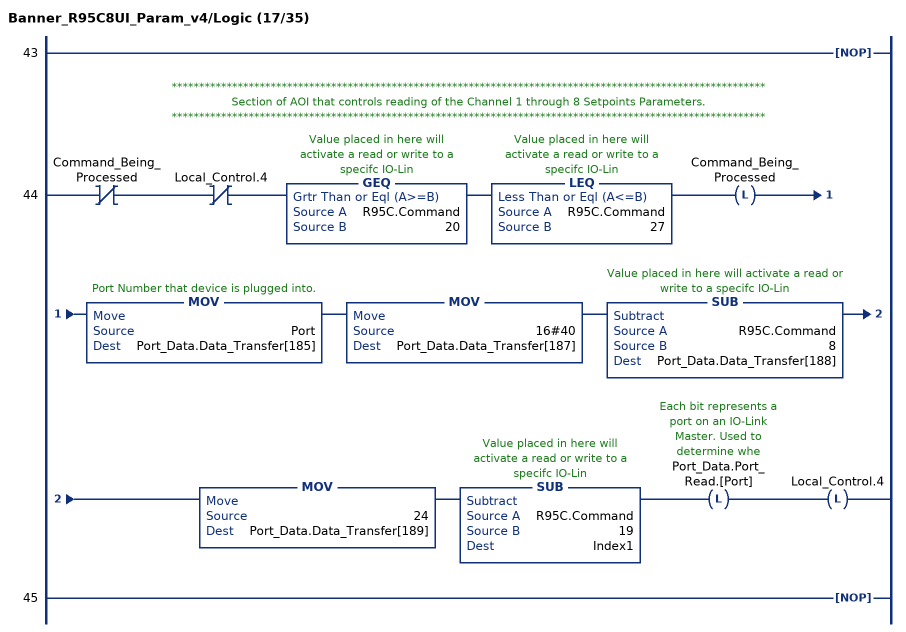
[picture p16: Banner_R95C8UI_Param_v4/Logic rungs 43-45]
   43: NOP();
   // ************************************************************************************************************
   // Section of AOI that controls reading of the Channel 1 through 8 Setpoints Parameters.
   // ************************************************************************************************************
   44: XIO(Command_Being_Processed)XIO(Local_Control.4)GEQ(R95C.Command,20)LEQ(R95C.Command,27)OTL(Command_Being_Processed)MOV(Port,Port_Data.Data_Transfer[185])MOV(16#40,Port_Data.Data_Transfer[187])SUB(R95C.Command,8,Port_Data.Data_Transfer[188])MOV(24,Port_Data.Data_Transfer[189])SUB(R95C.Command,19,Index1)OTL(Port_Data.Port_Read.[Port])OTL(Local_Control.4);
   45: NOP();
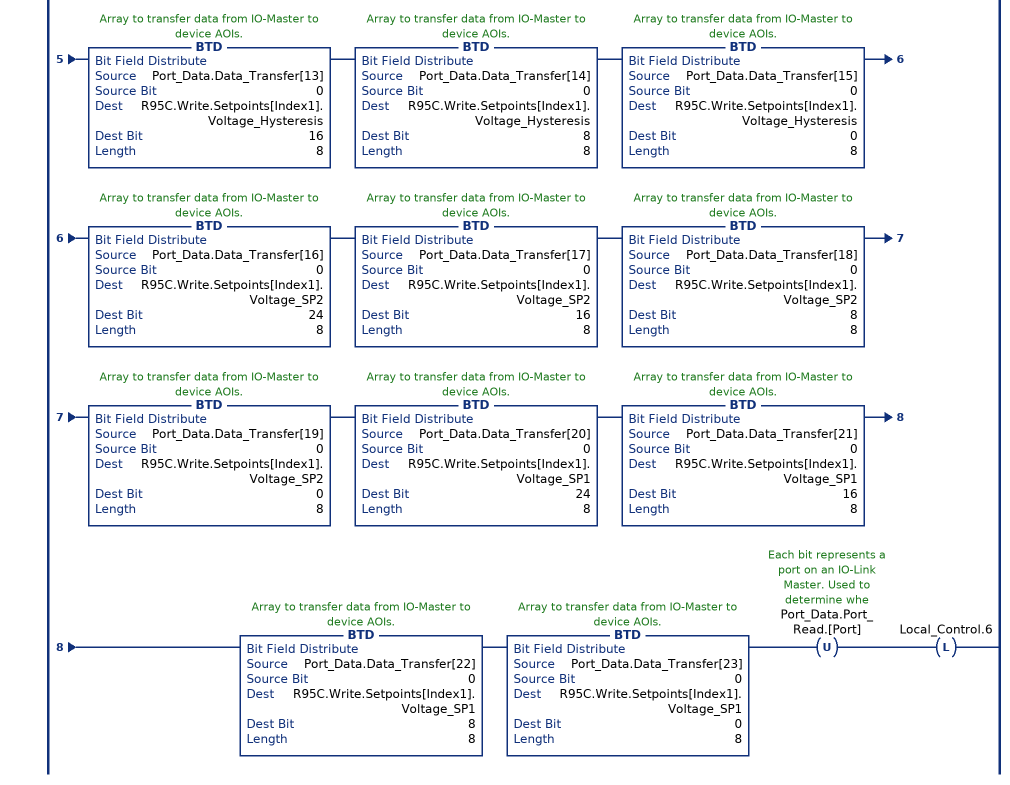
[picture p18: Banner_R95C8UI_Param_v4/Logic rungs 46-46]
   // Channel Setpoints Read data break out code.
   46: XIC(Local_Control.5)XIO(Local_Control.6)GEQ(R95C.Command,20)LEQ(R95C.Command,27)BTD(Port_Data.Data_Transfer[0],0,R95C.Write.Setpoints[Index1].Current_Hysteresis,24,8)BTD(Port_Data.Data_Transfer[1],0,R95C.Write.Setpoints[Index1].Current_Hysteresis,16,8)BTD(Port_Data.Data_Transfer[2],0,R95C.Write.Setpoints[Index1].Current_Hysteresis,8,8)BTD(Port_Data.Data_Transfer[3],0,R95C.Write.Setpoints[Index1].Current_Hysteresis,0,8)BTD(Port_Data.Data_Transfer[4],0,R95C.Write.Setpoints[Index1].Current_SP2,24,8)BTD(Port_Data.Data_Transfer[5],0,R95C.Write.Setpoints[Index1].Current_SP2,16,8)BTD(Port_Data.Data_Transfer[6],0,R95C.Write.Setpoints[Index1].Current_SP2,8,8)BTD(Port_Data.Data_Transfer[7],0,R95C.Write.Setpoints[Index1].Current_SP2,0,8)BTD(Port_Data.Data_Transfer[8],0,R95C.Write.Setpoints[Index1].Current_SP1,24,8)BTD(Port_Data.Data_Transfer[9],0,R95C.Write.Setpoints[Index1].Current_SP1,16,8)BTD(Port_Data.Data_Transfer[10],0,R95C.Write.Setpoints[Index1].Current_SP1,8,8)BTD(Port_Data.Data_Transfer[11],0,R95C.Write.Setpoints[Index1].Current_SP1,0,8)BTD(Port_Data.Data_Transfer[12],0,R95C.Write.Setpoints[Index1].Voltage_Hysteresis,24,8)BTD(Port_Data.Data_Transfer[13],0,R95C.Write.Setpoints[Index1].Voltage_Hysteresis,16,8)BTD(Port_Data.Data_Transfer[14],0,R95C.Write.Setpoints[Index1].Voltage_Hysteresis,8,8)BTD(Port_Data.Data_Transfer[15],0,R95C.Write.Setpoints[Index1].Voltage_Hysteresis,0,8)BTD(Port_Data.Data_Transfer[16],0,R95C.Write.Setpoints[Index1].Voltage_SP2,24,8)BTD(Port_Data.Data_Transfer[17],0,R95C.Write.Setpoints[Index1].Voltage_SP2,16,8)BTD(Port_Data.Data_Transfer[18],0,R95C.Write.Setpoints[Index1].Voltage_SP2,8,8)BTD(Port_Data.Data_Transfer[19],0,R95C.Write.Setpoints[Index1].Voltage_SP2,0,8)BTD(Port_Data.Data_Transfer[20],0,R95C.Write.Setpoints[Index1].Voltage_SP1,24,8)BTD(Port_Data.Data_Transfer[21],0,R95C.Write.Setpoints[Index1].Voltage_SP1,16,8)BTD(Port_Data.Data_Transfer[22],0,R95C.Write.Setpoints[Index1].Voltage_SP1,8,8)BTD(Port_Data.Data_Transfer[23],0,R95C.Write.Setpoints[Index1].Voltage_SP1,0,8)OTU(Port_Data.Port_Read.[Port])OTL(Local_Control.6);
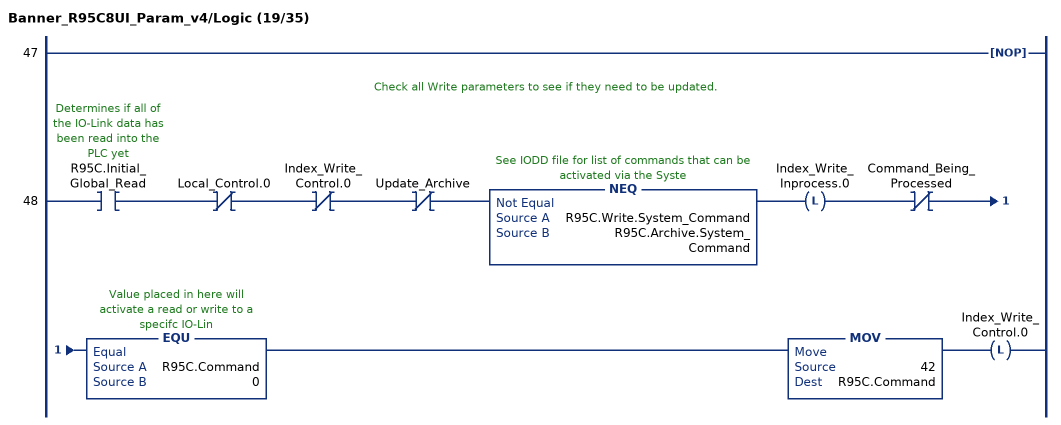
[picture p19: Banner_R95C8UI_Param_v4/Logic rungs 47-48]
   47: NOP();
   // Check all Write parameters to see if they need to be updated.
   48: XIC(R95C.Initial_Global_Read)XIO(Local_Control.0)XIO(Index_Write_Control.0)XIO(Update_Archive)NEQ(R95C.Write.System_Command,R95C.Archive.System_Command)OTL(Index_Write_Inprocess.0)XIO(Command_Being_Processed)EQU(R95C.Command,0)MOV(42,R95C.Command)OTL(Index_Write_Control.0);
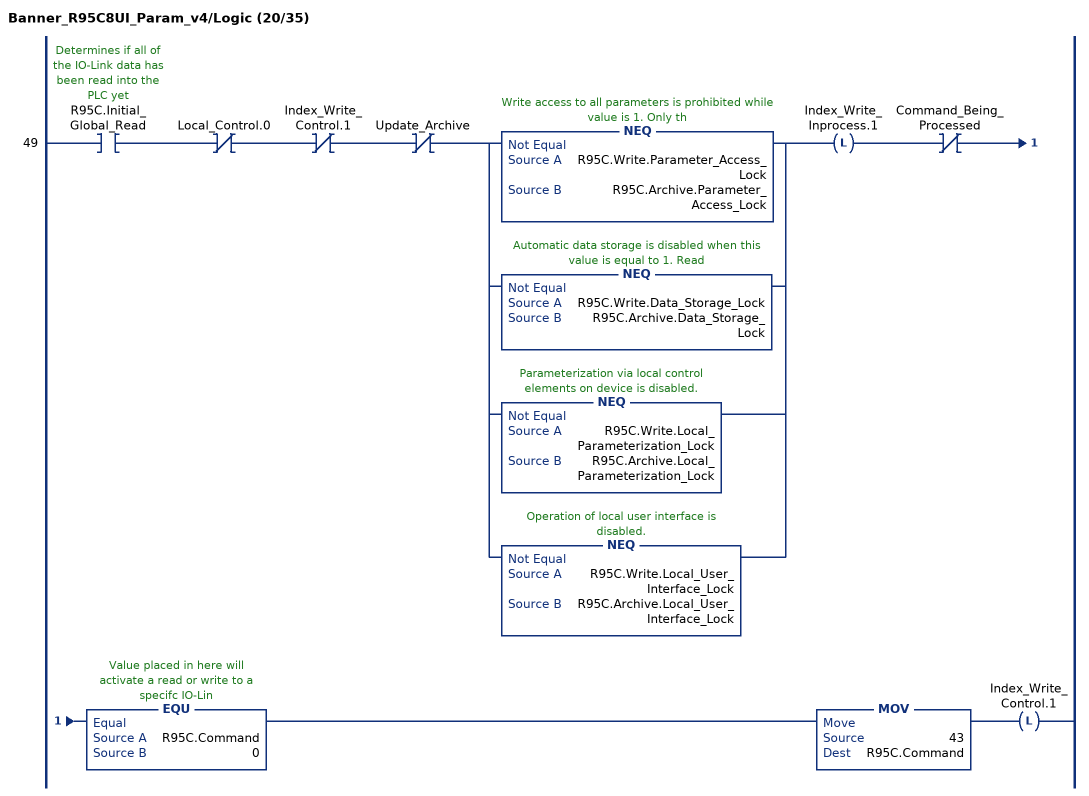
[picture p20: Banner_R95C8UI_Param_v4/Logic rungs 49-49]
   49: XIC(R95C.Initial_Global_Read)XIO(Local_Control.0)XIO(Index_Write_Control.1)XIO(Update_Archive)[NEQ(R95C.Write.Parameter_Access_Lock,R95C.Archive.Parameter_Access_Lock) ,NEQ(R95C.Write.Data_Storage_Lock,R95C.Archive.Data_Storage_Lock) ,NEQ(R95C.Write.Local_Parameterization_Lock,R95C.Archive.Local_Parameterization_Lock) ,NEQ(R95C.Write.Local_User_Interface_Lock,R95C.Archive.Local_User_Interface_Lock) ]OTL(Index_Write_Inprocess.1)XIO(Command_Being_Processed)EQU(R95C.Command,0)MOV(43,R95C.Command)OTL(Index_Write_Control.1);
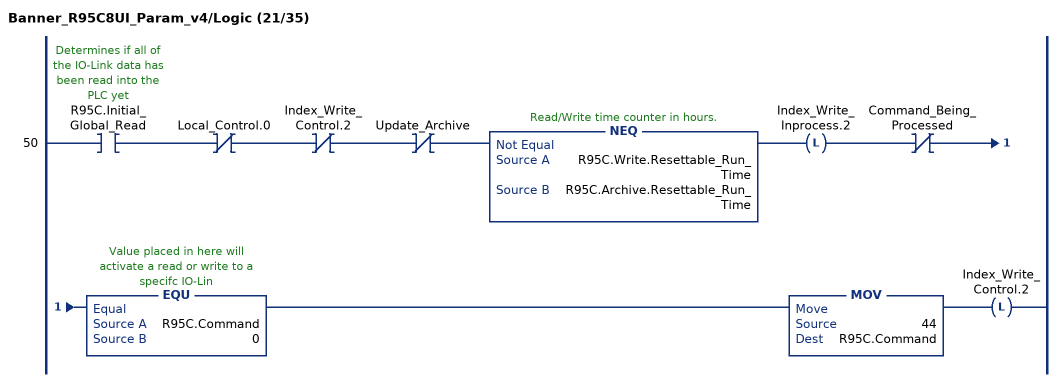
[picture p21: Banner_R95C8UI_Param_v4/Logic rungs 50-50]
   50: XIC(R95C.Initial_Global_Read)XIO(Local_Control.0)XIO(Index_Write_Control.2)XIO(Update_Archive)NEQ(R95C.Write.Resettable_Run_Time,R95C.Archive.Resettable_Run_Time)OTL(Index_Write_Inprocess.2)XIO(Command_Being_Processed)EQU(R95C.Command,0)MOV(44,R95C.Command)OTL(Index_Write_Control.2);
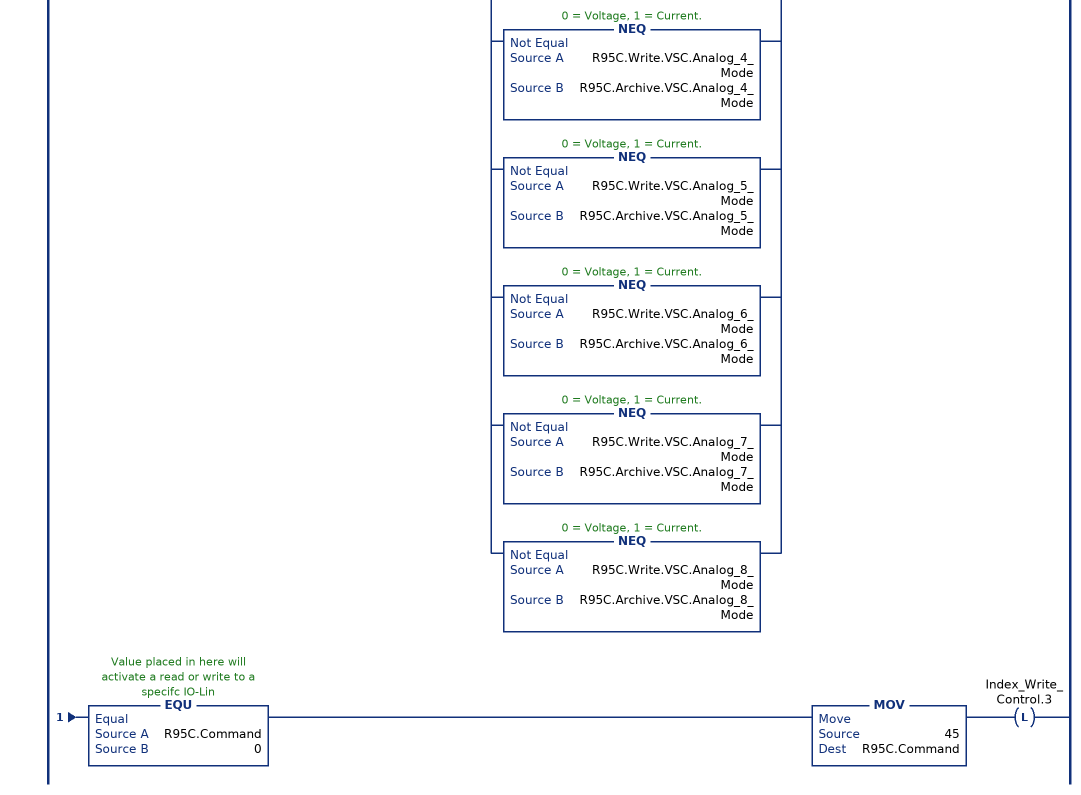
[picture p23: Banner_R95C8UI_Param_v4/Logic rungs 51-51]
   51: XIC(R95C.Initial_Global_Read)XIO(Local_Control.0)XIO(Index_Write_Control.3)XIO(Update_Archive)[NEQ(R95C.Write.VSC.PDI_Config,R95C.Archive.VSC.PDI_Config) ,NEQ(R95C.Write.VSC.IOL_Filter_Time,R95C.Archive.VSC.IOL_Filter_Time) ,NEQ(R95C.Write.VSC.Secondary_Output_Function,R95C.Archive.VSC.Secondary_Output_Function) ,NEQ(R95C.Write.VSC.PFM_Input_Port,R95C.Archive.VSC.PFM_Input_Port) ,NEQ(R95C.Write.VSC.Analog_1_Mode,R95C.Archive.VSC.Analog_1_Mode) ,NEQ(R95C.Write.VSC.Analog_2_Mode,R95C.Archive.VSC.Analog_2_Mode) ,NEQ(R95C.Write.VSC.Analog_3_Mode,R95C.Archive.VSC.Analog_3_Mode) ,NEQ(R95C.Write.VSC.Analog_4_Mode,R95C.Archive.VSC.Analog_4_Mode) ,NEQ(R95C.Write.VSC.Analog_5_Mode,R95C.Archive.VSC.Analog_5_Mode) ,NEQ(R95C.Write.VSC.Analog_6_Mode,R95C.Archive.VSC.Analog_6_Mode) ,NEQ(R95C.Write.VSC.Analog_7_Mode,R95C.Archive.VSC.Analog_7_Mode) ,NEQ(R95C.Write.VSC.Analog_8_Mode,R95C.Archive.VSC.Analog_8_Mode) ]OTL(Index_Write_Inprocess.3)XIO(Command_Being_Processed)EQU(R95C.Command,0)MOV(45,R95C.Command)OTL(Index_Write_Control.3);
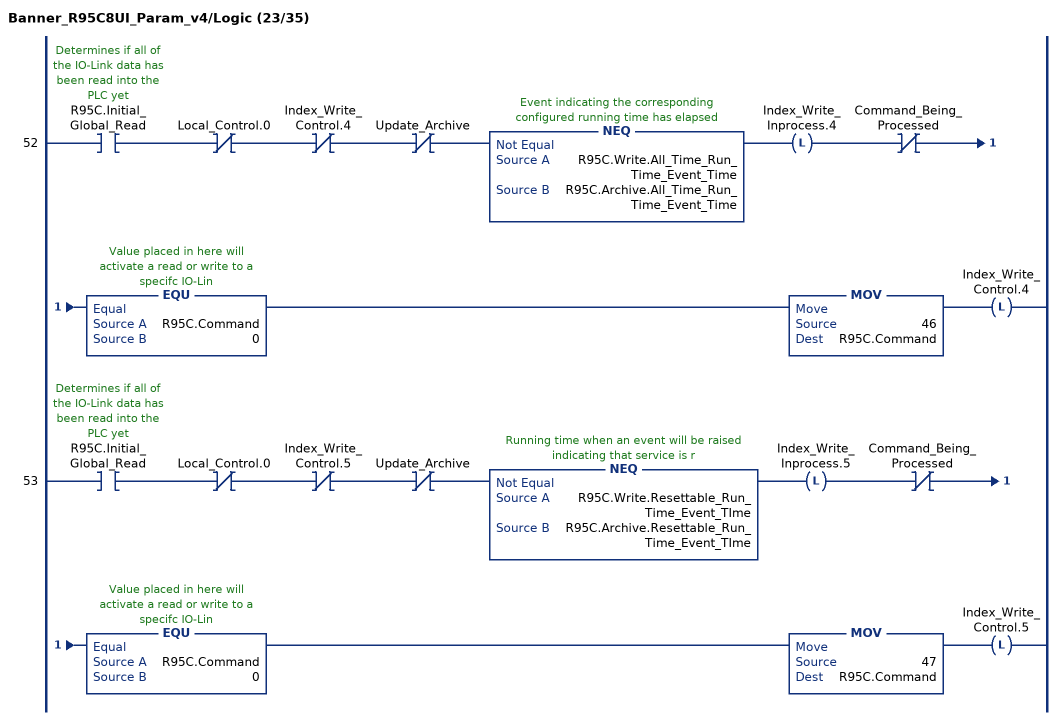
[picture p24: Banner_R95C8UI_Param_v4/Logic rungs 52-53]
   52: XIC(R95C.Initial_Global_Read)XIO(Local_Control.0)XIO(Index_Write_Control.4)XIO(Update_Archive)NEQ(R95C.Write.All_Time_Run_Time_Event_Time,R95C.Archive.All_Time_Run_Time_Event_Time)OTL(Index_Write_Inprocess.4)XIO(Command_Being_Processed)EQU(R95C.Command,0)MOV(46,R95C.Command)OTL(Index_Write_Control.4);
   53: XIC(R95C.Initial_Global_Read)XIO(Local_Control.0)XIO(Index_Write_Control.5)XIO(Update_Archive)NEQ(R95C.Write.Resettable_Run_Time_Event_TIme,R95C.Archive.Resettable_Run_Time_Event_TIme)OTL(Index_Write_Inprocess.5)XIO(Command_Being_Processed)EQU(R95C.Command,0)MOV(47,R95C.Command)OTL(Index_Write_Control.5);
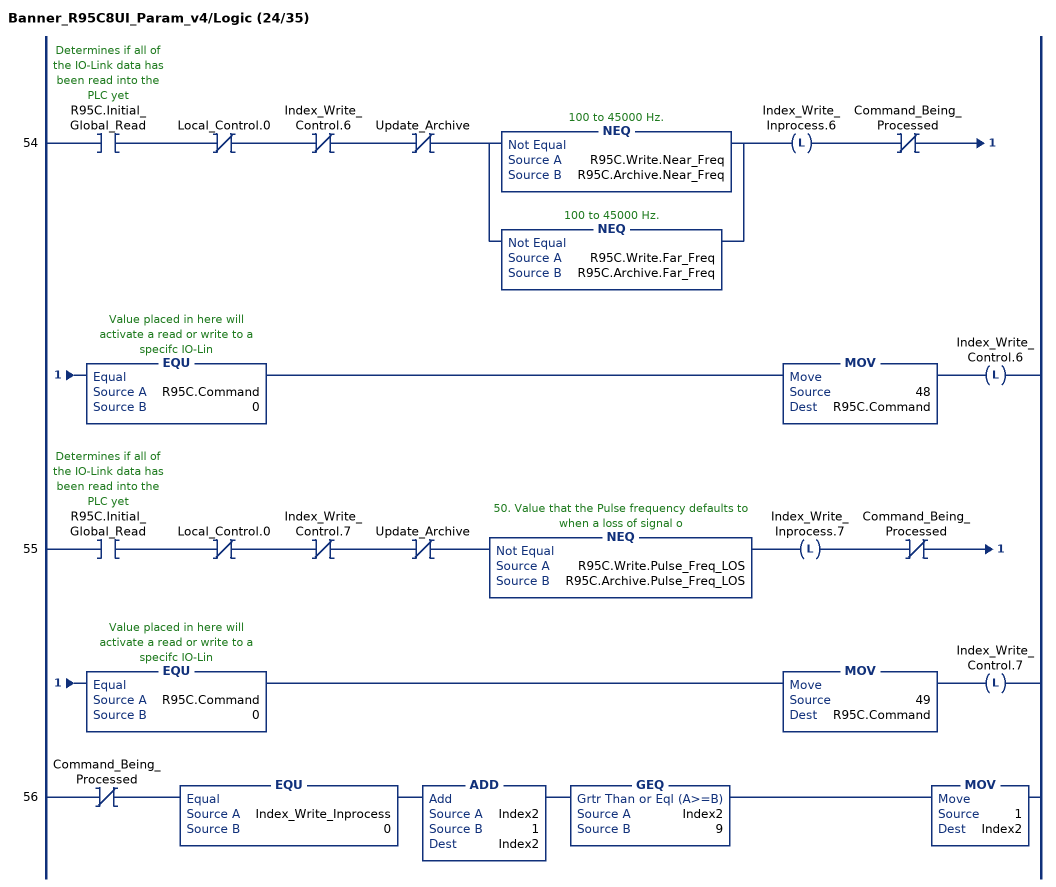
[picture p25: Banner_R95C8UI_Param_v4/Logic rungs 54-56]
   54: XIC(R95C.Initial_Global_Read)XIO(Local_Control.0)XIO(Index_Write_Control.6)XIO(Update_Archive)[NEQ(R95C.Write.Near_Freq,R95C.Archive.Near_Freq) ,NEQ(R95C.Write.Far_Freq,R95C.Archive.Far_Freq) ]OTL(Index_Write_Inprocess.6)XIO(Command_Being_Processed)EQU(R95C.Command,0)MOV(48,R95C.Command)OTL(Index_Write_Control.6);
   55: XIC(R95C.Initial_Global_Read)XIO(Local_Control.0)XIO(Index_Write_Control.7)XIO(Update_Archive)NEQ(R95C.Write.Pulse_Freq_LOS,R95C.Archive.Pulse_Freq_LOS)OTL(Index_Write_Inprocess.7)XIO(Command_Being_Processed)EQU(R95C.Command,0)MOV(49,R95C.Command)OTL(Index_Write_Control.7);
   56: XIO(Command_Being_Processed)EQU(Index_Write_Inprocess,0)ADD(Index2,1,Index2)GEQ(Index2,9)MOV(1,Index2);
